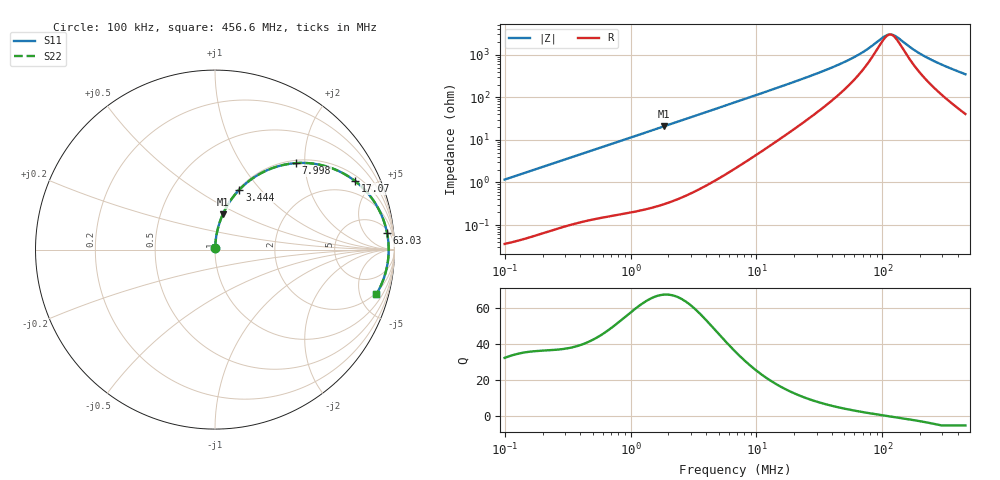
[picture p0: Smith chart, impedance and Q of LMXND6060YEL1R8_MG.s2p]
! LMXND6060YEL1R8_MG  S-PARAMETER MODEL  ( General Type )
! Model Generated by TAIYO YUDEN Corporation (http://www.ty-top.com)
! Version 1.0
! TAIYO YUDEN Control No. 191025NI43SB-FBB
! Copyright(c) 2019 TAIYO YUDEN CO.,LTD. All Rights Reserved.
! Product Description (link to TY-COMPAS)
! https://ds.yuden.co.jp/TYCOMPAS/or/detail?pn=LMXND6060YEL1R8NMG&u=M
! Products Name : Inductors
! Characteristics :
!  Inductance : 1.8 uH , SRF(min) : 80 MHz , DC Resistance(max) : 0.0247 Ohm
!  Rated Current : Saturation :7200 mA , Temp Rise : 3900 mA
!  Case Size : 6.0 x 6.0 / 0.236 x 0.236 [mm/inch] , Thickness : 4.5 / 0.177 [mm/inch]
!  (Conditions: Temperature = 25 degC , DC Bias Current/Voltage = 0A / 0V)
! External Node Assignments :
!  1  o---GGG---o  2
! GND o---------o GND
! Frequency Range : 0.1MHz  -  456.598367MHz  [ 402 STEP ]
# MHz S RI R 50
! Freq[MHz].  S11 Real  S11 Imag  S21 Real  S21 Imag  S12 Real  S12 Imag  S22 Real  S22 Imag
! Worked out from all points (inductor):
!   401 points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, 100 kHz to 456.6 MHz, reference 50 ohm
!   read as one part in series: L = 1.85 uH near 104.3 kHz
!   highest Q = 67.5 at 1.83 MHz (marker M1), where L = 1.8 uH
!   self-resonance near 115.4 MHz
!   S11 on the Smith chart (normalised r, x): 100 kHz: 1.00, +0.02; 3.444 MHz: 1.01, +0.78; 7.998 MHz: 1.06, +1.81; 17.07 MHz: 1.26, +3.92; 63.03 MHz: 7, +18; 456.6 MHz: 1.81, -6.93
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0.1  0.000496 0.0117  0.9995 -0.0117  0.9995 -0.0117  0.000496 0.0117
0.410178  0.00337 0.0467  0.9966 -0.0467  0.9966 -0.0467  0.00337 0.0467
0.894291  0.0119 0.0999  0.9881 -0.0999  0.9881 -0.0999  0.0119 0.0999
1.682457  0.0374 0.1823  0.9626 -0.1823  0.9626 -0.1823  0.0374 0.1823
1.830372  0.0436 0.197  0.9564 -0.197  0.9564 -0.197  0.0436 0.197
3.443534  0.1355 0.3337  0.8645 -0.3337  0.8645 -0.3337  0.1355 0.3337
4.823761  0.2336 0.4126  0.7664 -0.4126  0.7664 -0.4126  0.2336 0.4126
6.901063  0.3818 0.4719  0.6182 -0.4719  0.6182 -0.4719  0.3818 0.4719
7.997567  0.4521 0.4819  0.5479 -0.4819  0.5479 -0.4819  0.4521 0.4819
11.20313  0.6139 0.4654  0.3861 -0.4654  0.3861 -0.4654  0.6139 0.4654
17.07324  0.7791 0.383  0.2209 -0.383  0.2209 -0.383  0.7791 0.383
27.71655  0.8917 0.2602  0.1083 -0.2602  0.1083 -0.2602  0.8917 0.2602
44.05686  0.9416 0.1567  0.0584 -0.1567  0.0584 -0.1567  0.9416 0.1567
63.02949  0.959 0.0916  0.041 -0.0916  0.041 -0.0916  0.959 0.0916
77.80941  0.9642 0.058  0.0358 -0.058  0.0358 -0.058  0.9642 0.058
102.3215  0.9674 0.0174  0.0326 -0.0174  0.0326 -0.0174  0.9674 0.0174
113.6871  0.9677 0.00216  0.0323 -0.00216  0.0323 -0.00216  0.9677 0.00216
129.0043  0.9675 -0.0161  0.0325 0.0161  0.0325 0.0161  0.9675 -0.0161
176.9444  0.9636 -0.0631  0.0364 0.0631  0.0364 0.0631  0.9636 -0.0631
232.6867  0.9555 -0.1081  0.0445 0.1081  0.0445 0.1081  0.9555 -0.1081
325.9515  0.9361 -0.172  0.0639 0.172  0.0639 0.172  0.9361 -0.172
456.5984  0.8995 -0.2478  0.1005 0.2478  0.1005 0.2478  0.8995 -0.2478
